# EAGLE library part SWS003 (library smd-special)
SMD Dip Switch 3 pol.
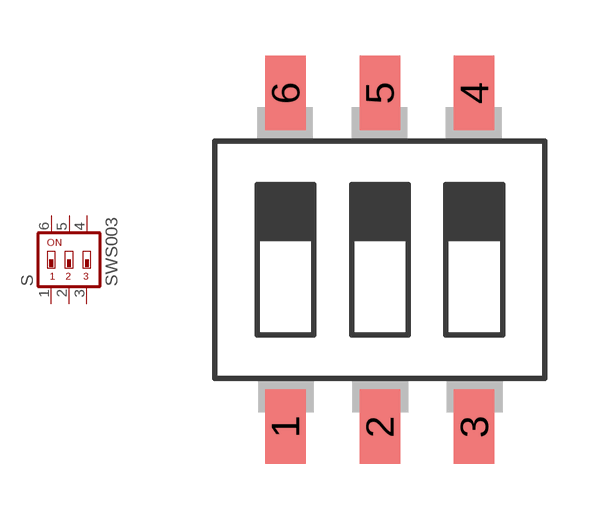
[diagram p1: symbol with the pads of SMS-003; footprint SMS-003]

Designator prefix S

## SWS003  [SMS-003]
1  1  pas
2  2  pas
3  3  pas
4  4  pas
5  5  pas
6  6  pas

## Footprint SMS-003 (pad centres in mm)
DIP SWITCH
smd 1.092 x 2.007: 1 -2.54,-4.496; 2 0,-4.496; 3 2.54,-4.496; 4 2.54,4.496; 5 0,4.496; 6 -2.54,4.496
